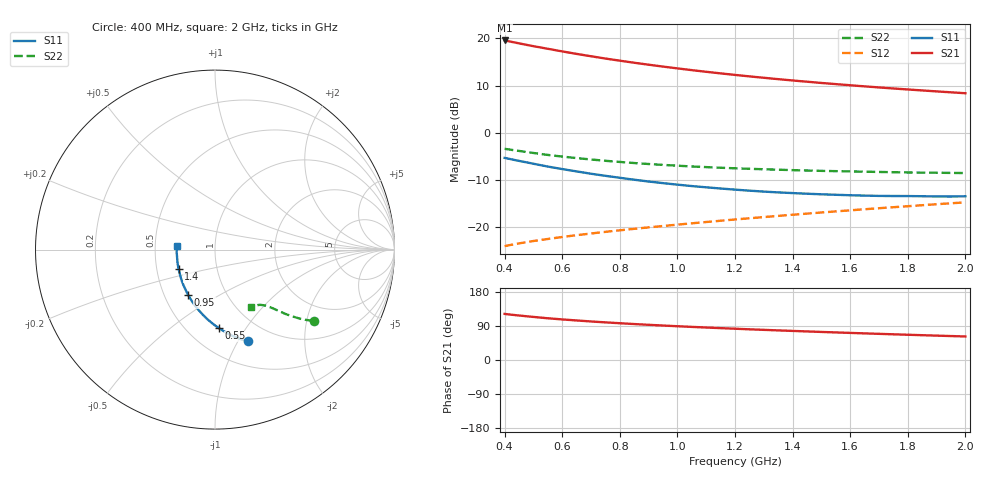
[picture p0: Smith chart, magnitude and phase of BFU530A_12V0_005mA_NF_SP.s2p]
! Filename:  P:\Prog\Test\Noise\ATS_data\Testdata_Net\06 Compressed Noise after Statistics\BFU530A_APG2013_33_A05_12p0V_005mA_NF_CM01_D.sf
! Date/Time: Tue 16/Apr/2013 15:10:59
! BFU530A_APG2013_33_A05_12p0V_1to25mA_NF_CM01_Bias4_R.sf
! Noise Parameter Data File
! BFU530A_APG2013_33_A05_12p0V_1to25mA_NF_CM01
! Date/time: Fri Apr 12 17:55:00 2013
! VAR V_out= 12.001000
! VAR I_out= 4.995000
! VAR V_in= 0.805700
! VAR I_in= 0.042600
! Device data file deembeded for feedlines and parallel
! Original file: \06 Compressed Noise after Statistics\BFU530A_APG2013_33_A05_12p0V_005mA_NF_CM01_R.sf
! Feed-files: PR017V01_150413_Feed1.s2p, PR017V01_150413_Feed2.s2p
! Parallel-file: PR017V01_150413_Par.s2p
# MHz S MA R 50
!  Freq-MHz  S11-mag  S11-arg  S21-mag  S21-arg  S12-mag  S12-arg  S22-mag  S22-arg
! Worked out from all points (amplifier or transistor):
!   37 points, 400 MHz to 2 GHz, reference 50 ohm
!   highest |S21| = 19.5 dB at 400 MHz (marker M1)
!   |S21| within 3 dB of that: start of sweep to 665.6 MHz
!   unconditionally stable (mu >= 1): 1.652 GHz to end of sweep
!   at 500 MHz: K = 0.59, MSG = 20.6 dB, |S12| = -22.9 dB
!   at 1.1 GHz: K = 0.91, MSG = 15.9 dB, |S12| = -18.9 dB
!   at 2 GHz: K = 1.01, MAG = 10.8 dB, |S12| = -14.7 dB
!   lowest NFmin = 0.62 dB at 420 MHz
!   S11 on the Smith chart (normalised r, x): 400 MHz: 0.76, -1.10; 550 MHz: 0.70, -0.76; 950 MHz: 0.66, -0.36; 1.4 GHz: 0.65, -0.15; 2 GHz: 0.65, +0.03
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400  0.5423 -70.2  9.478 121.6  0.06315 60.4  0.677 -35.8
420  0.5268 -72.7  9.212 119.8  0.065 60.0  0.6625 -36.6
440  0.5113 -75.1  8.96 118.2  0.0667 59.6  0.649 -37.2
480  0.4842 -79.5  8.47 115.1  0.06999 59.0  0.6233 -38.5
500  0.4704 -81.7  8.245 113.7  0.07161 58.7  0.6117 -39.0
550  0.4392 -87.0  7.74 110.1  0.07525 58.3  0.5829 -40.2
600  0.413 -91.8  7.259 107.1  0.07896 58.1  0.5599 -41.2
650  0.3902 -96.3  6.83 104.3  0.08257 58.0  0.5399 -42.1
700  0.3688 -100.7  6.451 101.7  0.08599 58.0  0.5217 -42.8
750  0.3504 -104.8  6.1 99.3  0.08948 58.1  0.5053 -43.4
800  0.3341 -109.0  5.792 97.0  0.09294 58.2  0.4916 -44.0
850  0.3187 -113.1  5.507 94.9  0.09633 58.4  0.4784 -44.5
900  0.3051 -117.0  5.25 92.9  0.09983 58.5  0.4674 -45.0
950  0.2933 -120.7  5.015 90.9  0.1032 58.8  0.4574 -45.6
1050  0.2731 -127.9  4.599 87.4  0.1102 59.3  0.4402 -46.4
1200  0.2504 -138.6  4.095 82.5  0.121 59.9  0.421 -47.9
1300  0.2387 -145.1  3.818 79.5  0.1283 60.3  0.4112 -48.9
1400  0.2302 -151.8  3.577 76.7  0.1358 60.6  0.4025 -50.0
1500  0.2235 -158.2  3.366 74.0  0.1434 60.8  0.3954 -51.2
1650  0.2164 -167.0  3.098 70.2  0.1552 61.0  0.3876 -53.1
1750  0.2142 -172.7  2.942 67.8  0.1631 61.1  0.3828 -54.3
2000  0.213 174.3  2.621 62.1  0.1837 61.0  0.375 -58.0
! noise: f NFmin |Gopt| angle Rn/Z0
400  0.6681  0.1913  20.9  0.1316
460  0.6675  0.1791  30.06  0.1186
600  0.7382  0.1772  32.31  0.135
800  0.7312  0.1575  57.04  0.11
1000  0.7421  0.1608  73.85  0.1023
1200  0.7981  0.1533  90.28  0.0991
1400  0.8395  0.1546  112.3  0.0914
1600  0.8535  0.1593  130.4  0.0838
1800  0.8323  0.2015  150.9  0.0697
2000  0.8705  0.1873  160.8  0.0769
